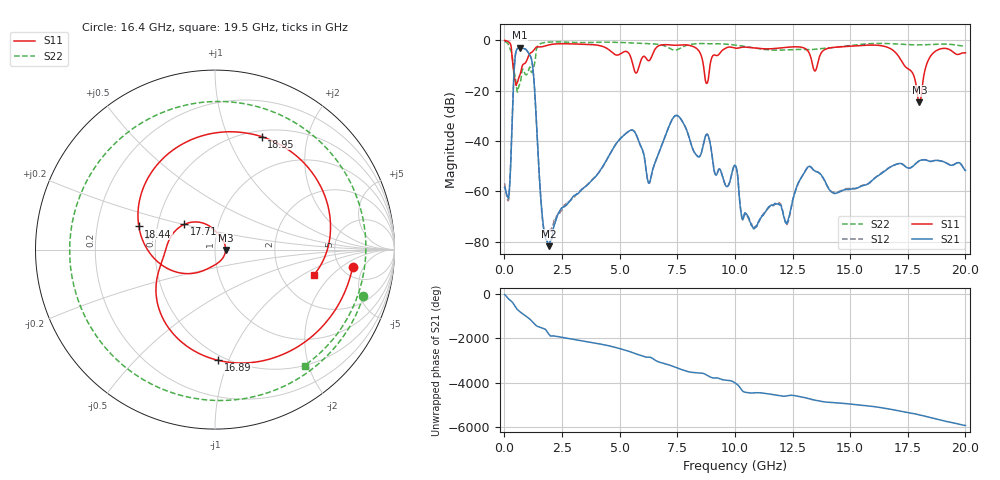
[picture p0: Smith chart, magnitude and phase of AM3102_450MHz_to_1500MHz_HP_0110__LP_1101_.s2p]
!Agilent Technologies,E8364B,MY43040894,A.07.50.67
!Agilent E8364B: A.07.50.67
!Date: Thursday, January 11, 2018 05:49:43
!Correction: S11(Full 2 Port(1,2))
!S21(Full 2 Port(1,2))
!S12(Full 2 Port(1,2))
!S22(Full 2 Port(1,2))
!S2P File: Measurements: S11, S21, S12, S22:
# Hz S  dB  R 50
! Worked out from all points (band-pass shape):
!   1601 points, 10 MHz to 20 GHz, reference 50 ohm
!   highest |S21| = -2.97 dB at 672.2 MHz (marker M1); lowest = -81.8 dB at 1.922 GHz (marker M2)
!   |S21| within 3 dB of the highest: 476.4 MHz to 1.107 GHz (630.7 MHz wide, 79.7 % of centre)
!   lowest |S11| = -24.6 dB at 18 GHz (marker M3), VSWR 1.13, Z = 56.3 - j0.309 ohm
!   |S11| at or under -10 dB: 371.2 MHz to 782.5 MHz (411.3 MHz wide, 71.3 % of centre); 8.635 GHz to 8.92 GHz (284.9 MHz wide, 3.25 % of centre); 17.35 GHz to 18.3 GHz (949.8 MHz wide, 5.33 % of centre)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
!   |S22| runs from -20.6 to -0.5 dB; largest |S21 - S12| = 0.0025
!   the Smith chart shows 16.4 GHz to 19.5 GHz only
!   S11 on the Smith chart (normalised r, x): 16.4 GHz: 6.29, -3.07; 16.89 GHz: 0.46, -0.92; 17.71 GHz: 0.68, +0.20; 18.44 GHz: 0.39, +0.13; 18.95 GHz: 0.57, +1.33; 19.5 GHz: 3.03, -1.28
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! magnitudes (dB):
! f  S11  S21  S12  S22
! 10 MHz  -0.1  -58.4  -56.8  -0.5
! 184.9 MHz  -0.6  -62.3  -63.4  -1.9
! 459.8 MHz  -15.9  -7.3  -7.3  -14.1
! 672.2 MHz  -13.9  -3.0  -3.0  -17.2
! 1.197 GHz  -4.7  -8.4  -8.4  -12.7
! 1.647 GHz  -2.5  -70.0  -70.9  -1.1
! 1.922 GHz  -1.9  -81.8  -76.0  -0.7
! 3.346 GHz  -1.6  -59.4  -59.3  -0.9
! 6.682 GHz  -2.2  -45.1  -45.2  -1.6
! 7.481 GHz  -2.0  -29.9  -29.9  -3.8
! 10.01 GHz  -3.1  -49.6  -49.7  -1.9
! 10.82 GHz  -3.1  -74.8  -74.6  -3.0
! 13.34 GHz  -8.6  -50.7  -50.8  -3.7
! 16.4 GHz  -2.2  -52.7  -52.5  -1.2
! 16.68 GHz  -3.0  -50.7  -50.7  -1.3
! 16.89 GHz  -4.2  -49.7  -49.7  -1.4
! 17.71 GHz  -13.1  -50.2  -50.1  -1.8
! 18 GHz  -24.6  -47.9  -47.9  -1.8
! 18.44 GHz  -7.1  -48.1  -48.0  -1.7
! 18.95 GHz  -3.3  -48.0  -48.0  -1.5
! 19.5 GHz  -4.9  -49.4  -49.4  -1.8
! 20 GHz  -5.0  -51.7  -51.8  -2.4
